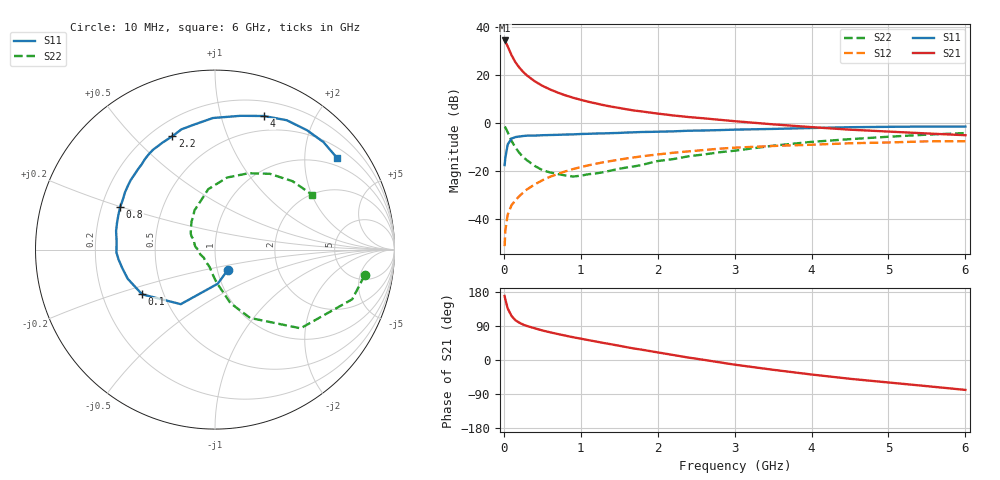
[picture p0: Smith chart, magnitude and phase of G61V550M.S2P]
! SIEMENS Small Signal Semiconductors
! BFG193
! Si NPN RF Bipolar Junction Transistor in SOT223
! VCE = 1.5 V  IC = 50 mA
! Common Emitter S-Parameters:  August  1996
# GHz  S  MA  R  50
!  f  S11  S21  S12  S22
! GHz  MAG  ANG  MAG  ANG  MAG  ANG  MAG  ANG
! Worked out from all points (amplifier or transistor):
!   36 points, 10 MHz to 6 GHz, reference 50 ohm
!   highest |S21| = 34.6 dB at 10 MHz (marker M1)
!   |S21| within 3 dB of that: start of sweep to 57.03 MHz
!   unconditionally stable (mu >= 1): 316.4 MHz to 2.745 GHz
!   at 250 MHz: K = 0.97, MSG = 25.2 dB, |S12| = -29.0 dB
!   at 1.4 GHz: K = 1.08, MAG = 9.6 dB, |S12| = -15.8 dB
!   at 6 GHz: K = 0.96, MSG = 1.3 dB, |S12| = -7.6 dB
!   S11 on the Smith chart (normalised r, x): 10 MHz: 1.12, -0.26; 100 MHz: 0.38, -0.24; 800 MHz: 0.28, +0.20; 2.2 GHz: 0.28, +0.65; 4 GHz: 0.34, +1.37; 6 GHz: 0.76, +2.80
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0.01  0.1333 -57.2  53.44 169.0  0.0027 87.3  0.8457 -9.8
0.02  0.1907 -85.4  50.6 159.6  0.0058 74.7  0.8131 -19.9
0.05  0.359 -122.1  40.13 136.1  0.0123 65.9  0.6479 -42.6
0.1  0.4767 -148.5  26.36 116.3  0.0194 62.8  0.4281 -62.8
0.15  0.5126 -161.5  18.8 105.0  0.0245 62.0  0.3103 -73.9
0.2  0.5264 -168.6  14.6 98.6  0.0298 64.6  0.2422 -79.2
0.25  0.5398 -174.0  11.82 93.5  0.0353 65.8  0.1954 -85.2
0.3  0.5494 -178.2  9.948 89.8  0.0413 66.6  0.1687 -89.5
0.4  0.5503 175.0  7.546 83.8  0.0524 67.0  0.1287 -97.9
0.5  0.5609 169.3  6.051 78.0  0.0641 66.0  0.1048 -105.5
0.6  0.566 164.6  5.072 73.2  0.0759 65.1  0.0937 -113.4
0.8  0.5791 155.9  3.817 64.3  0.0985 61.6  0.0809 -134.2
1.1  0.6005 144.3  2.798 52.4  0.1317 56.1  0.0859 -161.6
1.3  0.6124 137.6  2.375 44.8  0.1535 51.9  0.0949 -179.3
1.6  0.6375 127.8  1.942 33.7  0.184 44.6  0.1189 164.5
2.2  0.6748 110.6  1.452 13.3  0.241 30.3  0.1776 139.0
2.8  0.7168 95.4  1.178 -6.0  0.2929 15.7  0.2466 117.6
3.5  0.7589 79.2  0.946 -25.8  0.3343 -2.2  0.3385 96.4
4  0.7926 69.9  0.827 -38.3  0.3546 -12.0  0.407 80.5
4.5  0.8242 61.0  0.732 -49.6  0.3812 -22.1  0.4641 66.4
5.5  0.8508 44.8  0.61 -69.0  0.4178 -45.0  0.5762 41.4
6  0.8503 37.1  0.561 -78.9  0.419 -58.0  0.6222 29.3
